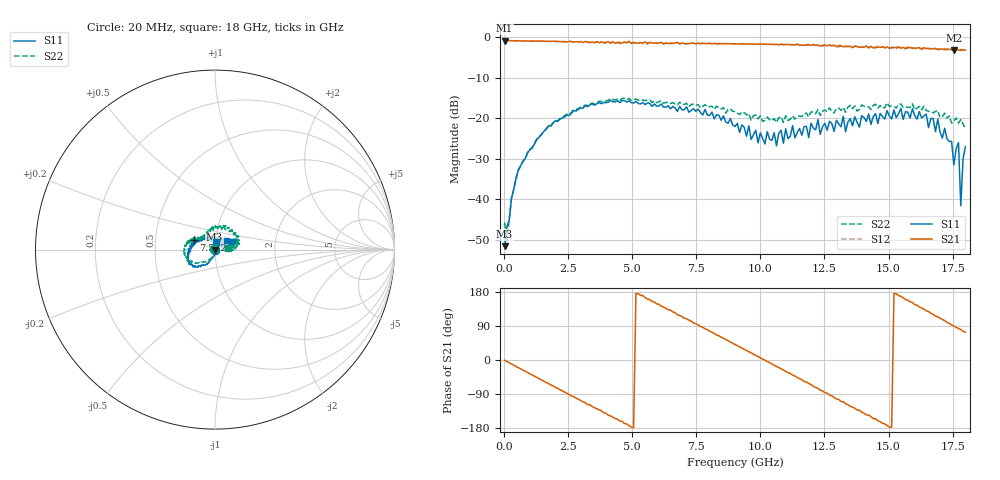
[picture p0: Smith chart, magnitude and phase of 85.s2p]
!Agilent Technologies,N5230A,US43500223,A.07.50.48
!Agilent N5230A: A.07.50.48
!Date: Sunday, January 31, 2016 15:14:46
!Correction: S11(Full 2 Port(1,2))
!S21(Full 2 Port(1,2))
!S12(Full 2 Port(1,2))
!S22(Full 2 Port(1,2))
!S2P File: Measurements: S11, S21, S12, S22:
# Hz S  RI  R 50
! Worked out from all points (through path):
!   201 points, 20 MHz to 18 GHz, reference 50 ohm
!   highest |S21| = -0.81 dB at 20 MHz (marker M1); lowest = -3.2 dB at 17.55 GHz (marker M2)
!   group delay of S21, straight-line fit = 99.3 ps
!   lowest |S11| = -51.5 dB at 20 MHz (marker M3), VSWR 1.01, Z = 49.7 - j0.0305 ohm
!   |S11| at or under -10 dB: start of sweep to end of sweep
!   |S22| runs from -50.2 to -15.1 dB; largest |S21 - S12| = 0.065
!   S11 on the Smith chart (normalised r, x): 20 MHz: 0.99, -0.00; 7.572 GHz: 0.78, +0.08; 18 GHz: 1.00, +0.09
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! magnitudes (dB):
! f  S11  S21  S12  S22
! 20 MHz  -51.5  -0.8  -0.8  -45.7
! 109.9 MHz  -46.8  -0.8  -0.8  -50.2
! 289.7 MHz  -39.7  -0.9  -0.9  -39.7
! 919 MHz  -28.5  -0.9  -0.9  -28.4
! 3.077 GHz  -17.5  -1.3  -1.2  -17.3
! 6.043 GHz  -16.9  -1.4  -1.6  -15.9
! 7.572 GHz  -17.7  -1.4  -1.4  -16.6
! 9.01 GHz  -22.0  -1.6  -1.6  -18.3
! 10.63 GHz  -26.8  -1.8  -1.7  -21.0
! 10.81 GHz  -22.9  -1.7  -1.8  -19.6
! 10.9 GHz  -26.1  -1.9  -1.8  -21.0
! 10.99 GHz  -22.6  -1.8  -1.8  -19.4
! 12.07 GHz  -22.4  -1.8  -1.9  -18.5
! 15.03 GHz  -19.4  -2.7  -2.7  -17.1
! 16.83 GHz  -23.3  -2.7  -2.9  -18.3
! 16.92 GHz  -20.2  -3.1  -2.9  -18.1
! 17.46 GHz  -25.7  -3.0  -3.1  -21.2
! 17.55 GHz  -31.5  -3.2  -3.2  -20.6
! 17.73 GHz  -26.0  -3.2  -3.2  -21.2
! 17.82 GHz  -41.6  -3.1  -3.3  -20.3
! 17.91 GHz  -30.0  -3.1  -3.2  -21.4
! 18 GHz  -27.0  -3.2  -3.3  -22.6
